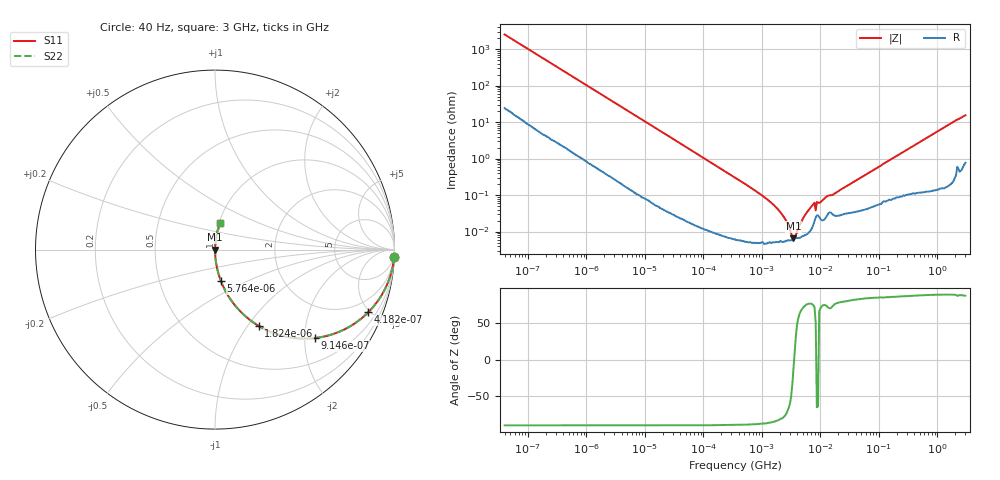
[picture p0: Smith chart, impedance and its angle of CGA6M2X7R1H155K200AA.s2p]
! S-parameter Generated by TDK Corporation
! Copyright(C) 2015 TDK Corporation.
! All Rights Reserved.
! TDK P/N: CGA6M2X7R1H155K200AA (Multilayer Ceramic Chip Capacitors)
! Property: C=1.5uF
! Size(LxWxT): 3.2x2.5x2mm, 0.126x0.098x0.079inches
! Model Type: s2p (Touchstone File Format Version 1.0)
! Frequency: DC=Yes Start=0.00004MHz Stop=3000MHz 396points Log-sweep
! Note: This model was converted from impedance.
! Model Generated on Jun. 23, 2015
! Hash(MD5):
! Port Assignments:
!  1 ---| |--- 2
! Applicable Conditions:
!  Temperature = 25 degC
!  DC Bias Voltage = 0 V
!  Small Signal Operation
! Terms and conditions regarding TDK Simulation Models
! (1)This simulation model is being provided solely for informational purposes. Please refer to the specifications of the products in terms of detailed characteristics of such products.
! (2)In no event shall TDK Corporation of any of its subsidiaries be liable for any loss or damage arising, directly or indirectly,
!  From any information contained in this simulation model, including, but not limited to loss or damages arising from any inaccuracies, omissions or errors in connection with such information.
! (3)Any and all copyrights on this simulation model are owned by TDK Corporation.
!  Duplication or redistribution of this simulation model without prior written permission from TDK Corporation is prohibited.
! (4)This simulation model is subject to any modification or change without any prior notice.
! (5)Neither TDK Corporation nor any of its subsidiaries shall make any warranty, express or implied,
!  Including but not limited to the correctness, implied warranties of merchantability and fitness for a particular purpose with respect to this simulation models.
! (6)The use of this simulation model shall be deemed to have consented to the terms and conditions hereof.
# MHz S MA R 50
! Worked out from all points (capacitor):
!   395 points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, 40 Hz to 3 GHz, reference 50 ohm
!   read as one part in series: C = 1.59 uF near 41.88 Hz
!   lowest |Z| = 6.47 mohm at 3.459 MHz (marker M1)
!   series resonance near 3.54 MHz, so ESL is about 1.3 nH
!   S11 on the Smith chart (normalised r, x): 40 Hz: 1, -50; 418.2 Hz: 1.04, -4.87; 914.6 Hz: 1.02, -2.24; 1.824 kHz: 1.01, -1.13; 5.764 kHz: 1.00, -0.36; 3 GHz: 1.02, +0.31
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4e-05  0.9988 -2.3  0.03992 87.2  0.03992 87.2  0.9988 -2.3
0.0001451139  0.9887 -8.1  0.1417 81.4  0.1417 81.4  0.9887 -8.1
0.0004182353  0.9224 -22.2  0.3786 67.3  0.3786 67.3  0.9224 -22.2
0.000834128  0.7719 -39.0  0.6295 50.5  0.6295 50.5  0.7719 -39.0
0.0009145504  0.7427 -41.6  0.6636 48.0  0.6636 48.0  0.7427 -41.6
0.001823978  0.4892 -60.3  0.8683 29.3  0.8683 29.3  0.4892 -60.3
0.005763764  0.1765 -79.4  0.983 10.2  0.983 10.2  0.1765 -79.4
0.01739424  0.05976 -86.1  0.9977 3.4  0.9977 3.4  0.05976 -86.1
0.3464102  0.003027 -88.7  0.9999 0.2  0.9999 0.2  0.003027 -88.7
1.581893  0.000539 -84.5  0.9999 0.0  0.9999 0.0  0.000539 -84.5
2.393669  0.000245 -77.5  0.9999 0.0  0.9999 0.0  0.000245 -77.5
3.154924  9.001e-05 -49.8  0.9999 0.0  0.9999 0.0  9.001e-05 -49.8
3.459106  6.47e-05 -11.8  0.9999 0.0  0.9999 0.0  6.47e-05 -11.8
3.971241  9.715e-05 47.0  0.9999 -0.0  0.9999 -0.0  9.715e-05 47.0
4.998775  0.0002252 70.5  0.9999 -0.0  0.9999 -0.0  0.0002252 70.5
7.22376  0.0005172 75.6  0.9999 -0.0  0.9999 -0.0  0.0005172 75.6
7.920238  0.0006145 71.6  0.9998 -0.0  0.9998 -0.0  0.0006145 71.6
8.293268  0.0003785 50.3  0.9998 -0.0  0.9998 -0.0  0.0003785 50.3
8.683867  0.0006476 -64.7  0.9997 0.0  0.9997 0.0  0.0006476 -64.7
9.521122  0.0006043 65.6  0.9998 -0.0  0.9998 -0.0  0.0006043 65.6
150.6385  0.008948 84.7  0.9992 -0.5  0.9992 -0.5  0.008948 84.7
3000  0.1499 78.5  0.9812 -8.6  0.9812 -8.6  0.1499 78.5
